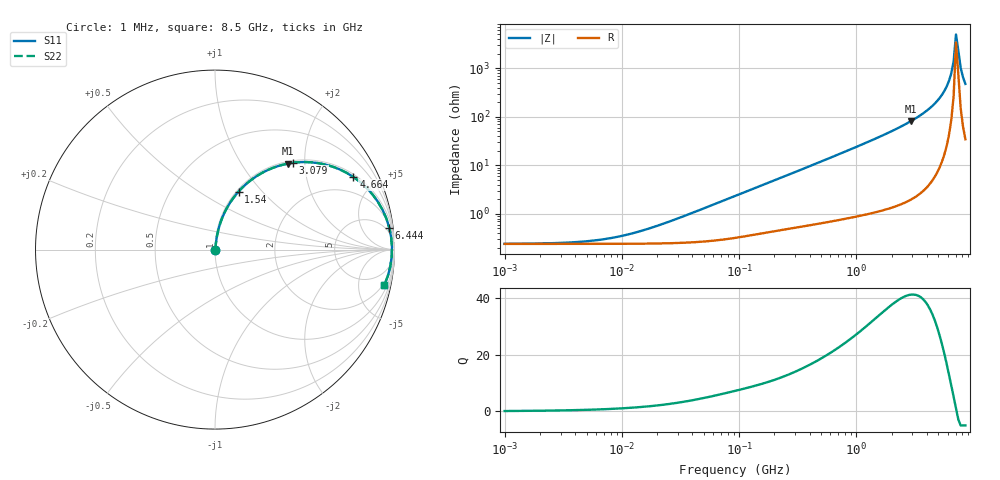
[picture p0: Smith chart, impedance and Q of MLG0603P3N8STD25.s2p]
! S-Parameter Data Generated by TDK Corporation
! Copyright(C) 2025 TDK Corporation.
! All Rights Reserved.
! TDK P/N: MLG0603P3N8STD25 (SMD / SMT Inductor (Coil))
! Property: L=3.8nH at 500MHz
! Size(LxWxT): 0.6x0.3x0.3mm
! Model Type: s2p (Touchstone File Format Version 1.0)
! Frequency: DC=Yes Start=1MHz Stop=8500MHz 198points Log-sweep
! Model Generated on Feb. 6, 2025
! Terms and conditions regarding TDK Simulation Models:
! 1)This simulation model is being provided solely for informational
!  purposes. Please refer to the specifications of the products in
!  terms of detailed characteristics of such products.
! 2)In no event shall TDK Corporation of any of its subsidiaries be
!  liable for any loss or damage arising, directly or indirectly,
!  from any information contained in this simulation model, including,
!  but not limited to loss or damages arising from any inaccuracies,
!  omissions or errors in connection with such information.
! 3)Any and all copyrights on this simulation model are owned by
!  TDK Corporation.  Duplication or redistribution of this simulation
!  model without prior written permission from TDK Corporation
!  is prohibited.
! 4)This simulation model is subject to any modification or change
!  without any prior notice.
! 5)Neither TDK Corporation nor any of its subsidiaries shall make any
!  warranty, express or implied, including but not limited to the
!  correctness, implied warranties of merchantability and fitness for
!  a particular purpose with respect to this simulation models.
! 6)The use of this simulation model shall be deemed to have consented
!  to the terms and conditions hereof.
! Port Assignments:
!  1 ---@@@--- 2
! Applicable Conditions:
!  Temperature = 25 degC
!  DC Bias Current = 0 A
!  Small Signal Operation
# Hz S MA R 50
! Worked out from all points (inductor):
!   197 points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, 1 MHz to 8.5 GHz, reference 50 ohm
!   read as one part in series: L = 4.05 nH near 30.45 MHz
!   highest Q = 41.3 at 2.94 GHz (marker M1), where L = 4.44 nH
!   self-resonance near 7.067 GHz
!   S11 on the Smith chart (normalised r, x): 1 MHz: 1.00, +0.00; 1.54 GHz: 1.02, +0.75; 3.079 GHz: 1.04, +1.75; 4.664 GHz: 1.12, +3.75; 6.444 GHz: 3, +16; 8.5 GHz: 1.69, -9.46
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1000000  0.002408 6.1  0.9976 -0.0  0.9976 -0.0  0.002408 6.1
4587603  0.002667 25.9  0.9976 -0.1  0.9976 -0.1  0.002667 25.9
9601846  0.003431 45.3  0.9976 -0.1  0.9976 -0.1  0.003431 45.3
2.10461e7  0.005889 65.1  0.9975 -0.3  0.9975 -0.3  0.005889 65.1
9.219544e7  0.02323 80.8  0.9966 -1.3  0.9966 -1.3  0.02323 80.8
4.229561e8  0.1003 80.9  0.9891 -5.7  0.9891 -5.7  0.1003 80.9
9.270694e8  0.2146 75.4  0.9685 -12.4  0.9685 -12.4  0.2146 75.4
1.540426e9  0.3492 67.9  0.9268 -20.4  0.9268 -20.4  0.3492 67.9
1.940355e9  0.4335 62.8  0.8896 -25.7  0.8896 -25.7  0.4335 62.8
2.939772e9  0.6266 49.8  0.7643 -38.8  0.7643 -38.8  0.6266 49.8
3.07866e9  0.6509 48.0  0.7436 -40.6  0.7436 -40.6  0.6509 48.0
3.877948e9  0.7761 37.6  0.6109 -50.9  0.6109 -50.9  0.7761 37.6
4.664383e9  0.8712 27.7  0.4647 -60.5  0.4647 -60.5  0.8712 27.7
5.115526e9  0.9122 22.2  0.3773 -65.7  0.3773 -65.7  0.9122 22.2
5.610304e9  0.946 16.3  0.2813 -70.9  0.2813 -70.9  0.946 16.3
6.152938e9  0.9705 10.2  0.1782 -75.4  0.1782 -75.4  0.9705 10.2
6.44363e9  0.9787 7.1  0.1247 -76.6  0.1247 -76.6  0.9787 7.1
6.748056e9  0.9839 4.0  0.07078 -74.9  0.07078 -74.9  0.9839 4.0
7.066863e9  0.9861 0.8  0.01992 -45.5  0.01992 -45.5  0.9861 0.8
7.750377e9  0.9813 -5.5  0.09664 76.1  0.09664 76.1  0.9813 -5.5
8.116539e9  0.9743 -8.6  0.1505 75.9  0.1505 75.9  0.9743 -8.6
8.5e9  0.9644 -11.7  0.2034 74.1  0.2034 74.1  0.9644 -11.7
